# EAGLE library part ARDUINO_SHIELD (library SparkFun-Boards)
Arduino shield footprint
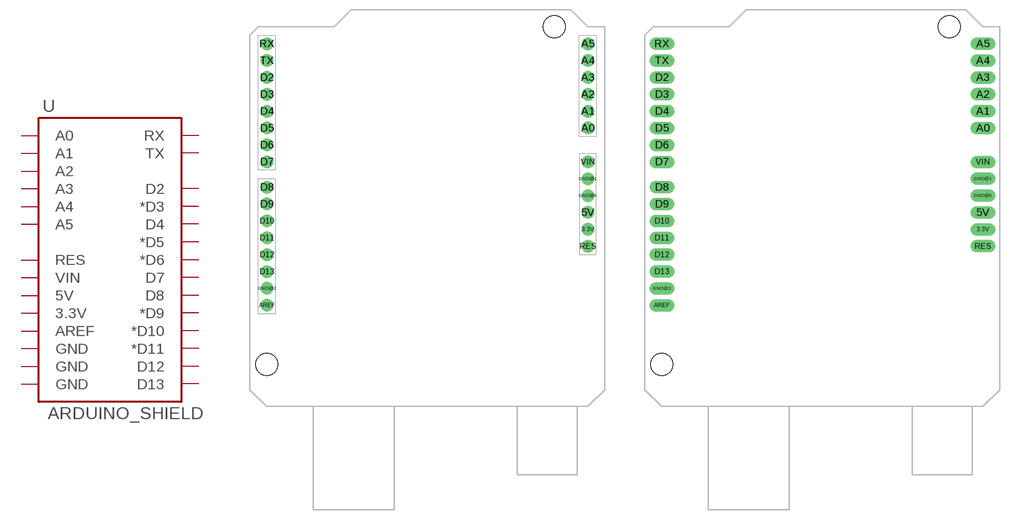
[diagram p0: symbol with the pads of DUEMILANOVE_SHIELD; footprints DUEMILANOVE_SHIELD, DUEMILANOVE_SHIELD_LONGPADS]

Designator prefix U

## ARDUINO_SHIELDLABEL  [DUEMILANOVE_SHIELD]
3.3V  3.3V
5V  5V
A0  A0
A1  A1
A2  A2
A3  A3
A4  A4
A5  A5
AREF  AREF
D2  D2
D3  *D3
D4  D4
D5  *D5
D6  *D6
D7  D7
D8  D8
D9  *D9
D10  *D10
D11  *D11
D12  D12
D13  D13
GND@0  GND
GND@1  GND
GND@2  GND
RES  RES
RX  RX
TX  TX
VIN  VIN

## ARDUINO_SHIELDLONGPADS  [DUEMILANOVE_SHIELD_LONGPADS]
Pads as for DUEMILANOVE_SHIELD

## ARDUINO_SHIELDNOHOLES  [DUEMILANOVE_SHIELD_NOHOLES]
Pads as for DUEMILANOVE_SHIELD

## ARDUINO_SHIELDNOHOLESORLABELS  [DUEMILANOVE_SHIELD_NOHOLES_NOLABELS]
Pads as for DUEMILANOVE_SHIELD

## ARDUINO_SHIELDNOLABELS  [DUEMILANOVE_SHIELD_NOLABELS]
Pads as for DUEMILANOVE_SHIELD

## ARDUINO_SHIELDNO_SILK  [DUEMILANOVE_VIAS]
Pads as for DUEMILANOVE_SHIELD

## Footprint DUEMILANOVE_SHIELD (pad centres in mm)
drill 1.016 pad 1.88: 3.3V 50.8,26.67; 5V 50.8,29.21; A0 50.8,41.91; A1 50.8,44.45; A2 50.8,46.99; A3 50.8,49.53; A4 50.8,52.07; A5 50.8,54.61; AREF 2.54,15.24; D2 2.54,49.53; D3 2.54,46.99; D4 2.54,44.45; D5 2.54,41.91; D6 2.54,39.37; D7 2.54,36.83; D8 2.54,33.02; D9 2.54,30.48; D10 2.54,27.94; D11 2.54,25.4; D12 2.54,22.86; D13 2.54,20.32; GND@0 50.8,31.75; GND@1 50.8,34.29; GND@2 2.54,17.78; RES 50.8,24.13; RX 2.54,54.61; TX 2.54,52.07; VIN 50.8,36.83
hole 3.302 at 45.72,57.15
hole 3.302 at 2.54,6.35

## Footprint DUEMILANOVE_SHIELD_LONGPADS (pad centres in mm)
drill 1.016 pad 1.88 long: 3.3V 50.8,26.67; 5V 50.8,29.21; A0 50.8,41.91; A1 50.8,44.45; A2 50.8,46.99; A3 50.8,49.53; A4 50.8,52.07; A5 50.8,54.61; AREF 2.54,15.24; D2 2.54,49.53; D3 2.54,46.99; D4 2.54,44.45; D5 2.54,41.91; D6 2.54,39.37; D7 2.54,36.83; D8 2.54,33.02; D9 2.54,30.48; D10 2.54,27.94; D11 2.54,25.4; D12 2.54,22.86; D13 2.54,20.32; GND@0 50.8,31.75; GND@1 50.8,34.29; GND@2 2.54,17.78; RES 50.8,24.13; RX 2.54,54.61; TX 2.54,52.07; VIN 50.8,36.83
hole 3.302 at 45.72,57.15
hole 3.302 at 2.54,6.35

## Footprint DUEMILANOVE_SHIELD_NOHOLES (pad centres in mm)
drill 1.016 pad 1.88: 3.3V 50.8,26.67; 5V 50.8,29.21; A0 50.8,41.91; A1 50.8,44.45; A2 50.8,46.99; A3 50.8,49.53; A4 50.8,52.07; A5 50.8,54.61; AREF 2.54,15.24; D2 2.54,49.53; D3 2.54,46.99; D4 2.54,44.45; D5 2.54,41.91; D6 2.54,39.37; D7 2.54,36.83; D8 2.54,33.02; D9 2.54,30.48; D10 2.54,27.94; D11 2.54,25.4; D12 2.54,22.86; D13 2.54,20.32; GND@0 50.8,31.75; GND@1 50.8,34.29; GND@2 2.54,17.78; RES 50.8,24.13; RX 2.54,54.61; TX 2.54,52.07; VIN 50.8,36.83

## Footprint DUEMILANOVE_SHIELD_NOHOLES_NOLABELS (pad centres in mm)
drill 1.016 pad 1.88: 3.3V 50.8,26.67; 5V 50.8,29.21; A0 50.8,41.91; A1 50.8,44.45; A2 50.8,46.99; A3 50.8,49.53; A4 50.8,52.07; A5 50.8,54.61; AREF 2.54,15.24; D2 2.54,49.53; D3 2.54,46.99; D4 2.54,44.45; D5 2.54,41.91; D6 2.54,39.37; D7 2.54,36.83; D8 2.54,33.02; D9 2.54,30.48; D10 2.54,27.94; D11 2.54,25.4; D12 2.54,22.86; D13 2.54,20.32; GND@0 50.8,31.75; GND@1 50.8,34.29; GND@2 2.54,17.78; RES 50.8,24.13; RX 2.54,54.61; TX 2.54,52.07; VIN 50.8,36.83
